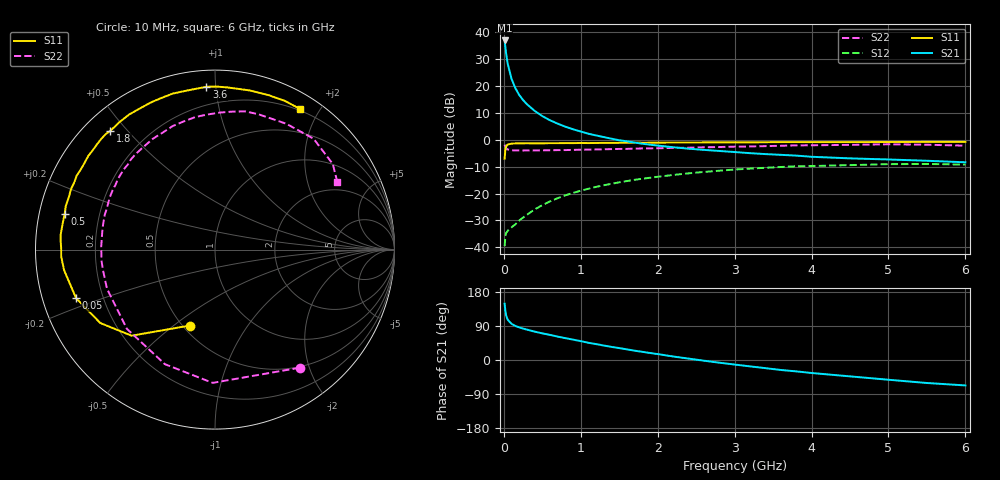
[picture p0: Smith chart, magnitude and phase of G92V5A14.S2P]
! SIEMENS Small Signal Semiconductors
! BFG235
! Si NPN RF Bipolar Junction Transistor in SOT223
! VCE = 2.5 V  IC = 140 mA
! Common Emitter S-Parameters:  July  1994
# GHz  S  MA  R  50
!  f  S11  S21  S12  S22
! GHz  MAG  ANG  MAG  ANG  MAG  ANG  MAG  ANG
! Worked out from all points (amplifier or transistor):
!   40 points, 10 MHz to 6 GHz, reference 50 ohm
!   highest |S21| = 37.0 dB at 10 MHz (marker M1)
!   |S21| within 3 dB of that: start of sweep to 22.03 MHz
!   unconditionally stable (mu >= 1): 434.6 MHz to 1.571 GHz
!   at 200 MHz: K = 0.81, MSG = 23.4 dB, |S12| = -30.0 dB
!   at 1.5 GHz: K = 1.01, MAG = 7.2 dB, |S12| = -15.8 dB
!   at 6 GHz: K = 0.92, MSG = 0.4 dB, |S12| = -9.2 dB
!   S11 on the Smith chart (normalised r, x): 10 MHz: 0.54, -0.57; 50 MHz: 0.10, -0.17; 500 MHz: 0.08, +0.12; 1.8 GHz: 0.08, +0.45; 3.6 GHz: 0.09, +0.94; 6 GHz: 0.18, +1.76
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0.01  0.446 -108.4  70.72 148.7  0.0105 59.1  0.8096 -54.4
0.02  0.6679 -134.1  52.91 129.0  0.0159 43.8  0.7426 -91.0
0.03  0.7589 -147.4  40.3 117.6  0.0184 37.2  0.6968 -113.6
0.05  0.8199 -160.7  26.17 106.2  0.0203 32.3  0.6602 -138.0
0.1  0.8485 -172.2  13.65 95.4  0.0235 35.7  0.64 -160.1
0.15  0.8578 -177.4  9.139 89.8  0.0268 42.3  0.6344 -169.3
0.2  0.8569 179.6  6.836 86.1  0.0315 47.2  0.6355 -174.5
0.25  0.8617 176.7  5.504 82.8  0.0358 50.9  0.6334 -178.3
0.3  0.8642 174.6  4.596 80.2  0.0403 54.1  0.6342 178.5
0.4  0.8611 170.1  3.463 74.9  0.0507 56.4  0.634 173.8
0.5  0.8611 166.6  2.766 70.3  0.0609 57.4  0.6374 169.7
0.7  0.8652 160.1  1.999 61.7  0.0821 56.7  0.6441 162.4
0.9  0.869 154.7  1.572 53.7  0.1031 53.9  0.6499 156.1
1.1  0.8709 148.3  1.298 45.4  0.1231 50.3  0.6594 149.9
1.4  0.8776 141.0  1.05 34.5  0.152 44.1  0.6726 141.2
1.8  0.8824 131.3  0.847 21.6  0.1887 35.3  0.6914 130.1
2.2  0.8919 122.4  0.729 9.3  0.2218 26.3  0.7079 119.3
3.2  0.8995 101.1  0.565 -16.8  0.2912 3.0  0.7535 93.4
3.6  0.9082 93.0  0.526 -26.3  0.3121 -6.7  0.7755 82.6
4.5  0.9077 77.6  0.452 -43.2  0.3384 -26.2  0.8061 60.4
5.5  0.9156 64.7  0.408 -60.7  0.3557 -47.6  0.8112 36.0
6  0.9155 58.7  0.382 -67.1  0.3459 -55.7  0.779 29.0
